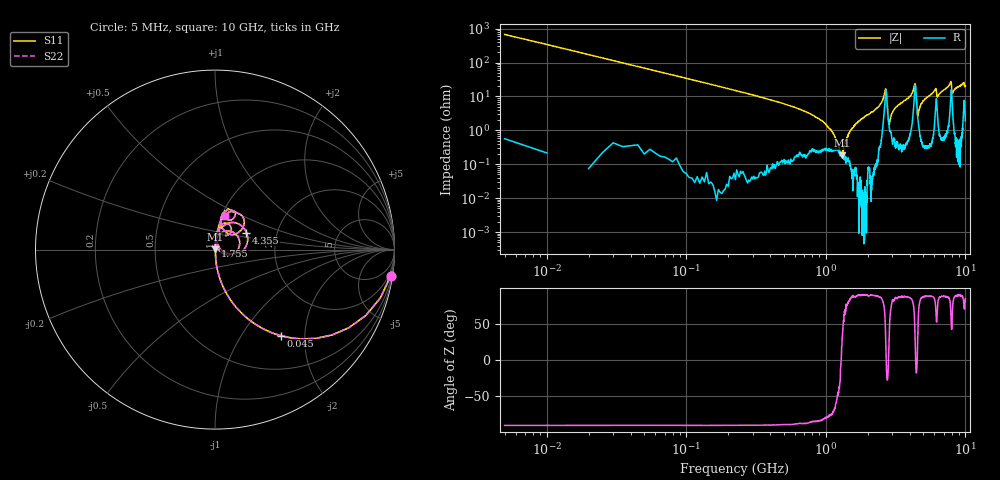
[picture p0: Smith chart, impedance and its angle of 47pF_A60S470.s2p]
! Amotech Co.,Ltd.
! http://www.amotech.co.kr/
! Part Number: A60S470
! These Parameters are Measured in Series Mode Connection
! Operation Temp=25[degC], DC Bias Voltage=0[V]
! Freq. Start=5[MHz] Stop=10[GHz], 2000[Steps]
! Date: Monday, July 13, 2020, 01:42:29
# GHZ S RI R 50.000000
!Freq.(Hz) S11(Real) S11(Imag) S21(Real) S21(Imag) S12(Real) S12(Imag) S22(Real) S22(Imag)
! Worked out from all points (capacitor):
!   2000 points, 5 MHz to 10 GHz, reference 50 ohm
!   read as one part in series: C = 46.2 pF near 55 MHz
!   lowest |Z| = 182 mohm at 1.3 GHz (marker M1)
!   series resonance near 1.287 GHz, so ESL is about 330 pH
!   S11 on the Smith chart (normalised r, x): 5 MHz: 1, -13; 45 MHz: 1.01, -1.53; 1.755 GHz: 1.00, +0.04; 4.355 GHz: 1.39, +0.28; 10 GHz: 1.04, +0.40
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0.005  0.9782 -0.1455  0.0218 0.1455  0.0218 0.1455  0.9782 -0.1455
0.045  0.3683 -0.4799  0.6317 0.4799  0.6317 0.4799  0.3683 -0.4799
0.1  0.1054 -0.3063  0.8946 0.3063  0.8946 0.3063  0.1054 -0.3063
0.19  0.0312 -0.1733  0.9688 0.1733  0.9688 0.1733  0.0312 -0.1733
0.97  0.00304 -0.0168  0.997 0.0168  0.997 0.0168  0.00304 -0.0168
1.3  0.00171 0.000614  0.9983 -0.000614  0.9983 -0.000614  0.00171 0.000614
1.48  0.00134 0.00875  0.9987 -0.00875  0.9987 -0.00875  0.00134 0.00875
1.675  0.000705 0.0166  0.9993 -0.0166  0.9993 -0.0166  0.000705 0.0166
1.755  0.000527 0.0199  0.9995 -0.0199  0.9995 -0.0199  0.000527 0.0199
2.665  0.0984 0.098  0.9016 -0.098  0.9016 -0.098  0.0984 0.098
2.85  0.0118 0.00935  0.9882 -0.00935  0.9882 -0.00935  0.0118 0.00935
3.34  0.00647 0.0569  0.9935 -0.0569  0.9935 -0.0569  0.00647 0.0569
4.355  0.1752 0.0952  0.8248 -0.0952  0.8248 -0.0952  0.1752 0.0952
4.56  0.0217 0.014  0.9783 -0.014  0.9783 -0.014  0.0217 0.014
5.005  0.00882 0.0738  0.9912 -0.0738  0.9912 -0.0738  0.00882 0.0738
6.105  0.0613 0.1479  0.9387 -0.1479  0.9387 -0.1479  0.0613 0.1479
6.29  0.0393 0.0845  0.9607 -0.0845  0.9607 -0.0845  0.0393 0.0845
6.67  0.0226 0.1279  0.9774 -0.1279  0.9774 -0.1279  0.0226 0.1279
7.845  0.1289 0.2029  0.8711 -0.2029  0.8711 -0.2029  0.1289 0.2029
8.05  0.0683 0.0927  0.9317 -0.0927  0.9317 -0.0927  0.0683 0.0927
8.335  0.0311 0.1507  0.9689 -0.1507  0.9689 -0.1507  0.0311 0.1507
10  0.0555 0.1862  0.9445 -0.1862  0.9445 -0.1862  0.0555 0.1862
